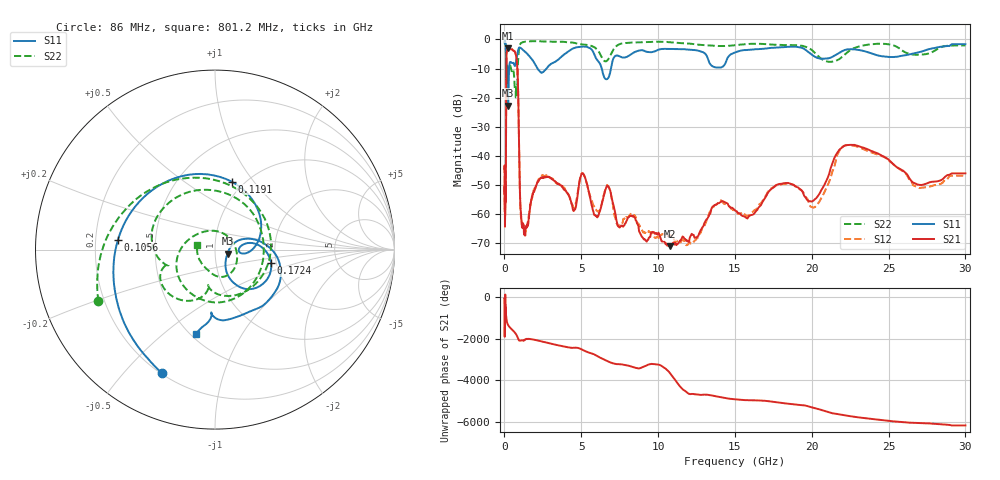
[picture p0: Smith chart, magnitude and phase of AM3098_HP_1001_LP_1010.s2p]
! Date/Time: Thu, Feb 28, 2019 8:41 AM
! Network Analyzer: Agilent Technologies E8364B Rev: A.07.50.67
! Sweep from 0.010 to 30.000 GHz, 1601 Points, Sweep Type: LOG
! Power Supply: 5.023 V, 0.002 A
# Hz S DB R 50
!freq MagS11 AngS11 MagS21 AngS21 MagS12 AngS12 MagS22 AngS22
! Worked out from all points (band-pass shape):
!   1601 points, 10 MHz to 30 GHz, reference 50 ohm
!   highest |S21| = -3.06 dB at 243.5 MHz (marker M1); lowest = -71.0 dB at 10.76 GHz (marker M2)
!   |S21| within 3 dB of the highest: 130.2 MHz to 770.7 MHz (640.5 MHz wide, 142 % of centre)
!   lowest |S11| = -22.7 dB at 239.9 MHz (marker M3), VSWR 1.16, Z = 57.4 - j2.58 ohm
!   |S11| at or under -10 dB: 191.6 MHz to 302.6 MHz (111 MHz wide, 44.9 % of centre); 2.155 GHz to 2.736 GHz (580.4 MHz wide, 23.7 % of centre); 6.335 GHz to 6.931 GHz (595.8 MHz wide, 8.98 % of centre)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
!   |S22| runs from -20.0 to -0.6 dB; largest |S21 - S12| = 0.011
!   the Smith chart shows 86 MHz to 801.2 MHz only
!   S11 on the Smith chart (normalised r, x): 86 MHz: 0.20, -0.64; 105.6 MHz: 0.30, +0.04; 119.1 MHz: 0.88, +0.78; 172.4 MHz: 1.87, -0.32; 801.2 MHz: 0.53, -0.65
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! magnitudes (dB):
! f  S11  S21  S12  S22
! 10 MHz  -0.3  -44.7  -44.1  -0.6
! 38.04 MHz  -0.5  -61.5  -60.5  -0.9
! 86 MHz  -2.5  -53.1  -51.4  -3.0
! 105.6 MHz  -5.3  -29.4  -29.4  -6.7
! 119.1 MHz  -8.2  -11.9  -11.9  -10.2
! 144.7 MHz  -17.2  -4.4  -4.3  -13.4
! 172.4 MHz  -9.8  -3.8  -3.8  -9.2
! 239.9 MHz  -22.7  -3.1  -3.0  -11.3
! 243.5 MHz  -22.4  -3.1  -3.0  -11.2
! 550.5 MHz  -8.0  -3.7  -3.7  -10.6
! 801.2 MHz  -6.4  -7.3  -7.3  -19.9
! 1.115 GHz  -3.2  -63.3  -62.6  -1.1
! 2.084 GHz  -9.3  -49.9  -49.7  -0.6
! 4.525 GHz  -3.0  -58.9  -57.9  -1.1
! 5.128 GHz  -2.4  -46.2  -46.2  -1.7
! 5.959 GHz  -6.5  -60.7  -58.5  -3.1
! 6.619 GHz  -13.7  -51.0  -50.9  -7.5
! 7.926 GHz  -6.1  -62.6  -61.0  -1.2
! 10.76 GHz  -3.3  -71.0  -67.6  -0.9
! 20.31 GHz  -6.2  -54.5  -57.1  -5.1
! 22.56 GHz  -3.4  -36.2  -36.4  -3.5
! 30 GHz  -1.6  -46.0  -46.8  -2.1
